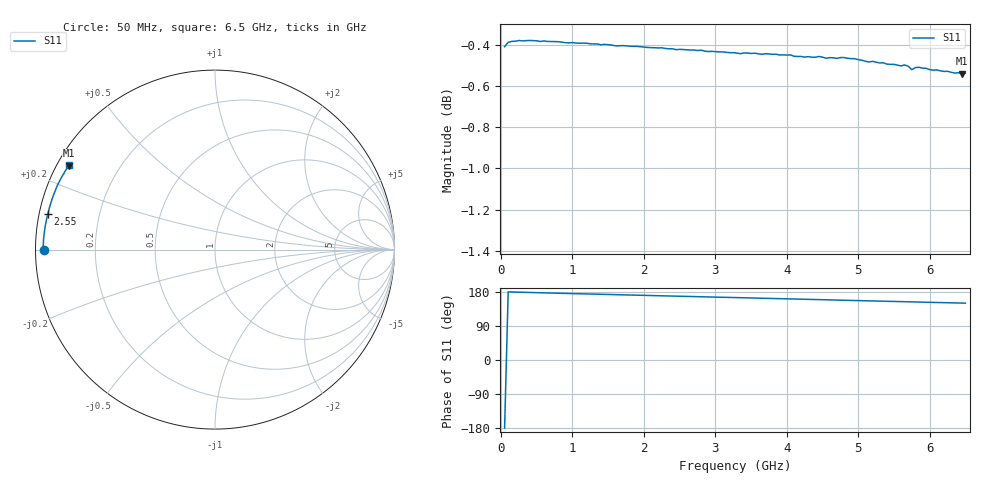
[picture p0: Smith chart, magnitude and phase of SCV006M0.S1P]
! Infineon Technologies  Discrete & RF Semiconductors
! BAR63-02L
! Si PIN Diode in TSLP-2
! IF = 6 mA
! S-Parameters:  March  2002
# GHz  S  MA  R  50
!  f  S11
! GHz  MAG  ANG
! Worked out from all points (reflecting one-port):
!   130 points, 50 MHz to 6.5 GHz, reference 50 ohm
!   lowest |S11| = -0.5 dB at 6.45 GHz (marker M1), VSWR 32.27, Z = 1.66 + j13.3 ohm
!   phase of S11 starts at -180 deg and turns -30 deg over the sweep
!   S11 on the Smith chart (normalised r, x): 50 MHz: 0.02, -0.00; 2.55 GHz: 0.02, +0.10; 6.5 GHz: 0.03, +0.27
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0.05  0.9541 -179.7
0.1  0.9565 179.9
0.2  0.957 179.2
0.9  0.9563 175.7
1.7  0.9547 172.0
1.75  0.9546 171.7
1.9  0.9543 171.1
2.25  0.9535 169.4
2.5  0.9527 168.3
2.55  0.9526 168.1
2.75  0.9521 167.1
3.25  0.9509 164.9
3.3  0.9507 164.6
3.6  0.9504 163.2
3.75  0.9503 162.6
4.1  0.949 160.9
4.25  0.9486 160.3
4.3  0.9488 160.0
4.55  0.9479 158.9
4.9  0.9477 157.2
5.15  0.946 156.0
5.3  0.9455 155.4
5.35  0.9456 155.1
5.7  0.9437 153.6
5.75  0.9419 153.4
5.9  0.9427 152.6
6.45  0.9399 150.2
6.5  0.9401 150.0
